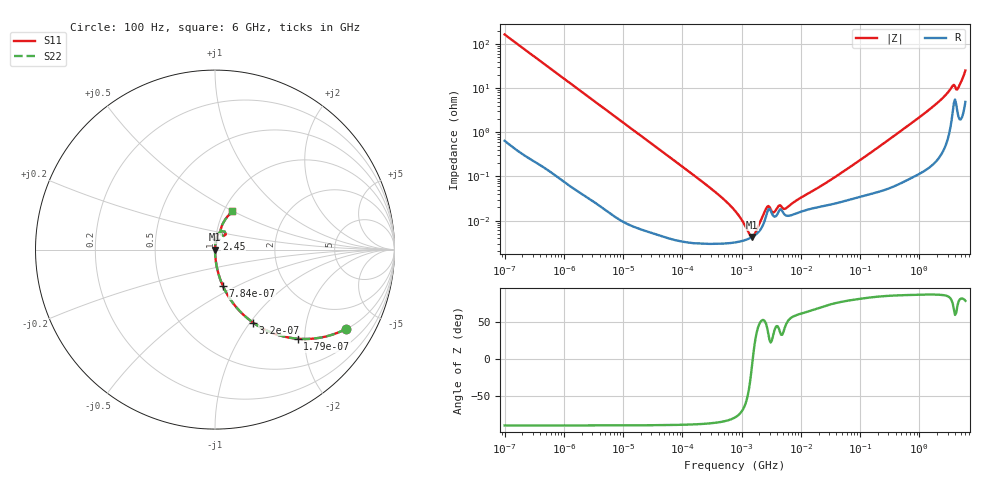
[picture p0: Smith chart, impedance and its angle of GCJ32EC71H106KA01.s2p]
!Murata Part Number: GCJ32EC71H106KA01
!These Parameters are Measured in Series Mode Connection
!Data Generated on Mar 13, 2026
!  o--ll--o
!Port1  Port2
!  o------o
!Operation Temp=25[degC], DC Bias Voltage=0[V]
!Freq. Start=100[Hz] Stop=6[GHz] 401[Steps]
# Hz S RI R 50
!Freq.(Hz) S11(Real) S11(Imag) S21(Real) S21(Imag) S12(Real) S12(Imag) S22(Real) S22(Imag)
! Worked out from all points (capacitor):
!   401 points, 100 Hz to 6 GHz, reference 50 ohm
!   read as one part in series: C = 9.63 uF near 109 Hz
!   lowest |Z| = 4.29 mohm at 1.516 MHz (marker M1)
!   series resonance near 1.545 MHz, so ESL is about 1.1 nH
!   S11 on the Smith chart (normalised r, x): 100 Hz: 1.01, -3.30; 179 Hz: 1.01, -1.85; 320 Hz: 1.00, -1.03; 784 Hz: 1.00, -0.42; 2.45 GHz: 1.01, +0.12; 6 GHz: 1.10, +0.49
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100  0.7307 -0.4417  0.2693 0.4417  0.2693 0.4417  0.7307 -0.4417
179  0.4604 -0.4965  0.5396 0.4965  0.5396 0.4965  0.4604 -0.4965
320  0.2117 -0.4064  0.7883 0.4064  0.7883 0.4064  0.2117 -0.4064
784  0.0437 -0.2021  0.9563 0.2021  0.9563 0.2021  0.0437 -0.2021
2008  0.00721 -0.0822  0.9928 0.0822  0.9928 0.0822  0.00721 -0.0822
40335  6.38e-05 -0.00416  0.9999 0.00416  0.9999 0.00416  6.38e-05 -0.00416
330837  2.99e-05 -0.000487  1 0.000487  1 0.000487  2.99e-05 -0.000487
774597  3.21e-05 -0.000165  1 0.000165  1 0.000165  3.21e-05 -0.000165
1059725  3.51e-05 -8.6e-05  1 8.6e-05  1 8.6e-05  3.51e-05 -8.6e-05
1516199  4.27e-05 -4.3e-06  1 4.3e-06  1 4.3e-06  4.27e-05 -4.3e-06
2074311  6.23e-05 7.41e-05  0.9999 -7.41e-05  0.9999 -7.41e-05  6.23e-05 7.41e-05
2713602  0.000155 0.000137  0.9998 -0.000137  0.9998 -0.000137  0.000155 0.000137
3394479  0.00013 7.88e-05  0.9999 -7.88e-05  0.9999 -7.88e-05  0.00013 7.88e-05
4246196  0.000162 0.000145  0.9998 -0.000145  0.9998 -0.000145  0.000162 0.000145
5554849  0.000132 0.000135  0.9999 -0.000135  0.9999 -0.000135  0.000132 0.000135
1.555665e7  0.000189 0.000424  0.9998 -0.000424  0.9998 -0.000424  0.000189 0.000424
5.211241e7  0.000274 0.00126  0.9997 -0.00126  0.9997 -0.00126  0.000274 0.00126
3.124326e8  0.000589 0.00694  0.9994 -0.00694  0.9994 -0.00694  0.000589 0.00694
2.450438e9  0.00688 0.0582  0.9931 -0.0582  0.9931 -0.0582  0.00688 0.0582
3.505958e9  0.0282 0.0978  0.9718 -0.0978  0.9718 -0.0978  0.0282 0.0978
4.586474e9  0.0316 0.0963  0.9684 -0.0963  0.9684 -0.0963  0.0316 0.0963
6e9  0.0967 0.2126  0.9033 -0.2126  0.9033 -0.2126  0.0967 0.2126
